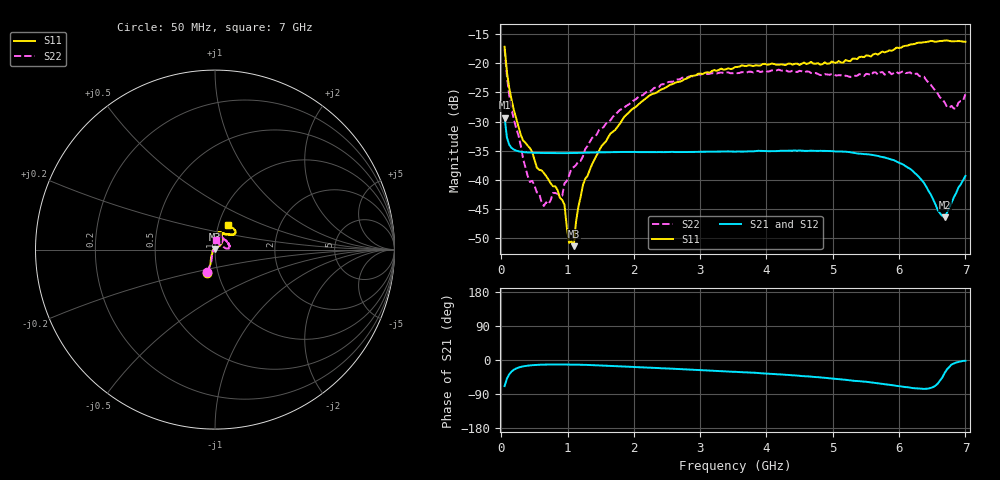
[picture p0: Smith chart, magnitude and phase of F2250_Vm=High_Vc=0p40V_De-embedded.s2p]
! Integrated Device Technology
! Corporate Headquarters
! 6024 Silver Creek Valley Road
! San Jose, CA 95138  USA
! Phone:  1-408-284-8200
! Toll Free:  1-800-223-1366
! Webpage:  http://www.idt.com/
! Timing and RF Division
! 515 Groton Road, Suite 102
! Westford, MA 01886-6024
! Device:  F2250
! Description: Voltage Variable RF Attenuator
! Frequency:  50.0 -  6000.00 MHz
! Package:  3x3 mm Thin QFN Plastic Package: 16 pin
! Ports:  2 RF, 3 DC
!  Pin  1  = GND
!  Pin  2  = NC
!  Pin  3  = RF1  = Port 1
!  Pin  4  = NC
!  Pin  5  = GND
!  Pin  6  = GND
!  Pin  7  = GND
!  Pin  8  = GND
!  Pin  9  = NC
!  Pin 10  = RF2  = Port 2
!  Pin 11  = NC
!  Pin 12  = GND
!  Pin 13  = GND
!  Pin 14  = VCNTRL
!  Pin 15  = VDD
!  Pin 16  = VMODE
! Vcntrl:  0.400 Volts
! Vmode:  +3.300 Volts
! Vdd:  +3.30  Volts
! Current:  1.264 mA
! Data:  The device was measured on a the F2250 evaluation board which has
!  individual transmission lines to the RF pins.  Data was collected
!  using a calibrated network analyzer.  The evaluation board was
!  de-embedded using a TRL calibration technique.
!  The reference plane is the edge of the package pin.
! Misc:  SN 10
!  Action Tracker AT0258
! Date Measured:  2014-11-26
! Date:  2015-10-15  MJV
! Note:
!  Integrated Device Technology supplies this data as a sample of measured
!  data at the package pin for this product.  Your particular data for this
!  product may vary.
!  Data was taken at 25 degrees C.
!  Integrated Device Technology reserves the right to change this data at anytime.
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# GHz S dB R 50
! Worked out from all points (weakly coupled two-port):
!   201 points, 50 MHz to 7 GHz, reference 50 ohm
!   highest |S21| = -29.32 dB at 50 MHz (marker M1); lowest = -46.4 dB at 6.687 GHz (marker M2)
!   lowest |S11| = -51.4 dB at 1.093 GHz (marker M3), VSWR 1.01, Z = 50 + j0.271 ohm
!   |S11| at or under -10 dB: start of sweep to end of sweep
!   |S22| runs from -44.5 to -17.6 dB; largest |S21 - S12| = 5.4e-05
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0.05  -17.18 -108.5  -29.32 -68.7  -29.32 -68.7  -17.62 -109.3
0.1195  -24.20 -112.0  -33.96 -37.8  -33.96 -37.8  -25.51 -109.8
0.29325  -32.26 -127.4  -35.17 -18.3  -35.16 -18.2  -34.08 -121.9
0.43225  -34.54 -145.3  -35.31 -14.2  -35.32 -14.2  -40.36 -158.4
0.5365  -37.89 -154.6  -35.36 -12.9  -35.36 -12.9  -42.14 -175.6
0.64075  -38.78 -162.6  -35.39 -12.2  -35.39 -12.2  -44.47 150.4
0.77975  -41.08 176.5  -35.41 -11.8  -35.41 -11.9  -42.25 122.5
0.91875  -43.44 155.9  -35.41 -11.9  -35.41 -11.9  -42.70 100.3
0.9535  -44.27 170.9  -35.41 -11.9  -35.41 -11.9  -40.58 101.2
1.023  -50.80 140.3  -35.40 -12.0  -35.40 -12.0  -39.26 83.1
1.0925  -51.35 89.8  -35.38 -12.1  -35.38 -12.2  -37.80 76.0
1.12725  -47.16 61.1  -35.38 -12.3  -35.37 -12.3  -37.46 68.8
1.2315  -40.86 40.8  -35.34 -12.6  -35.34 -12.6  -35.95 57.1
1.6485  -32.03 41.2  -35.26 -15.4  -35.26 -15.4  -29.75 50.2
2.37825  -24.75 46.7  -35.22 -21.3  -35.22 -21.4  -24.07 48.9
3.525  -20.65 71.7  -35.15 -31.1  -35.16 -31.1  -21.66 70.4
4.7065  -20.06 72.0  -35.00 -44.5  -35.00 -44.5  -21.71 68.9
5.85325  -17.79 40.5  -36.41 -65.3  -36.41 -65.4  -21.49 20.9
6.3745  -16.40 40.9  -40.49 -76.2  -40.51 -76.2  -22.30 4.7
6.68725  -16.11 47.8  -46.38 -34.3  -46.38 -34.1  -26.71 26.4
6.861  -16.22 54.5  -42.24 -6.6  -42.18 -6.5  -27.78 58.0
7  -16.32 62.4  -39.32 -2.2  -39.30 -2.5  -25.33 85.9
